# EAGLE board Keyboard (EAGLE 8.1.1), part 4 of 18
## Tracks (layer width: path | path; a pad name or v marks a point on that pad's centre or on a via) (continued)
S$3094 (continued)
  Bottom 0: 16.6,44.39 16.81,44.78
S$3095
  Bottom 0: 16.81,44.78 16.94,45.21
S$3096
  Bottom 0: 16.94,45.21 16.98,45.66
S$3097
  Bottom 0: 16.98,45.66 16.94,46.1
S$3098
  Bottom 0: 16.94,46.1 16.81,46.53
S$3099
  Bottom 0: 16.81,46.53 16.6,46.93
S$3100
  Bottom 0: 16.6,46.93 16.31,47.27
S$3101
  Bottom 0: 16.31,47.27 15.97,47.56
S$3102
  Bottom 0: 15.97,47.56 15.57,47.77
S$3103
  Bottom 0: 15.57,47.77 15.15,47.89
S$3104
  Bottom 0: 15.15,47.89 14.7,47.94
S$3105
  Bottom 0: 14.7,47.94 14.25,47.89
S$3106
  Bottom 0: 14.25,47.89 13.82,47.77
S$3107
  Bottom 0: 13.82,47.77 13.43,47.56
S$3108
  Bottom 0: 13.43,47.56 13.08,47.27
S$3109
  Bottom 0: 13.08,47.27 12.8,46.93
S$3110
  Bottom 0: 12.8,46.93 12.59,46.53
S$3111
  Bottom 0: 12.59,46.53 12.46,46.1
S$3112
  Bottom 0: 12.46,46.1 12.41,45.66
S$3113
  Bottom 0: 12.41,45.66 12.46,45.21
S$3114
  Bottom 0: 12.46,45.21 12.59,44.78
S$3115
  Bottom 0: 12.59,44.78 12.8,44.39
S$3116
  Bottom 0: 12.8,44.39 13.08,44.04
S$3117
  Bottom 0: 13.08,44.04 13.43,43.76
S$3118
  Bottom 0: 13.43,43.76 13.82,43.54
S$3119
  Bottom 0: 13.82,43.54 14.25,43.42
S$3120
  Bottom 0: 14.25,43.42 14.7,43.37
S$3121
  Bottom 0: 9.62,52.8 9.94,52.82
S$3122
  Bottom 0: 9.94,52.82 10.25,52.93
S$3123
  Bottom 0: 10.25,52.93 10.51,53.11
S$3124
  Bottom 0: 10.51,53.11 10.72,53.37
S$3125
  Bottom 0: 10.72,53.37 10.85,53.67
S$3126
  Bottom 0: 10.85,53.67 10.89,53.98
S$3127
  Bottom 0: 10.89,53.98 10.85,54.3
S$3128
  Bottom 0: 10.85,54.3 10.72,54.61
S$3129
  Bottom 0: 10.72,54.61 10.51,54.86
S$3130
  Bottom 0: 10.51,54.86 10.25,55.05
S$3131
  Bottom 0: 10.25,55.05 9.94,55.16
S$3132
  Bottom 0: 9.94,55.16 9.62,55.18
S$3133
  Bottom 0: 9.62,55.18 9.3,55.11
S$3134
  Bottom 0: 9.3,55.11 9.01,54.96
S$3135
  Bottom 0: 9.01,54.96 8.78,54.74
S$3136
  Bottom 0: 8.78,54.74 8.6,54.47
S$3137
  Bottom 0: 8.6,54.47 8.51,54.15
S$3138
  Bottom 0: 8.51,54.15 8.51,53.83
S$3139
  Bottom 0: 8.51,53.83 8.6,53.51
S$3140
  Bottom 0: 8.6,53.51 8.78,53.23
S$3141
  Bottom 0: 8.78,53.23 9.01,53.01
S$3142
  Bottom 0: 9.01,53.01 9.3,52.87
S$3143
  Bottom 0: 9.3,52.87 9.62,52.8
S$3144
  Bottom 0: 9.86,58.23 10.21,58.3
S$3145
  Bottom 0: 10.21,58.3 10.52,58.45
S$3146
  Bottom 0: 10.52,58.45 10.79,58.67
S$3147
  Bottom 0: 10.79,58.67 11,58.96
S$3148
  Bottom 0: 11,58.96 11.13,59.28
S$3149
  Bottom 0: 11.13,59.28 11.17,59.63
S$3150
  Bottom 0: 11.17,59.63 11.13,59.97
S$3151
  Bottom 0: 11.13,59.97 11,60.3
S$3152
  Bottom 0: 11,60.3 10.79,60.58
S$3153
  Bottom 0: 10.79,60.58 10.52,60.8
S$3154
  Bottom 0: 10.52,60.8 10.21,60.96
S$3155
  Bottom 0: 10.21,60.96 9.86,61.02
S$3156
  Bottom 0: 9.86,61.02 9.51,61
S$3157
  Bottom 0: 9.51,61 9.18,60.89
S$3158
  Bottom 0: 9.18,60.89 8.89,60.7
S$3159
  Bottom 0: 8.89,60.7 8.65,60.45
S$3160
  Bottom 0: 8.65,60.45 8.48,60.14
S$3161
  Bottom 0: 8.48,60.14 8.39,59.8
S$3162
  Bottom 0: 8.39,59.8 8.39,59.45
S$3163
  Bottom 0: 8.39,59.45 8.48,59.11
S$3164
  Bottom 0: 8.48,59.11 8.65,58.8
S$3165
  Bottom 0: 8.65,58.8 8.89,58.55
S$3166
  Bottom 0: 8.89,58.55 9.18,58.36
S$3167
  Bottom 0: 9.18,58.36 9.51,58.26
S$3168
  Bottom 0: 9.51,58.26 9.86,58.23
S$3169
  Bottom 0: 10.16,68.64 11.94,68.64
S$3170
  Bottom 0: 11.94,68.64 12.01,68.65
S$3171
  Bottom 0: 12.01,68.65 12.08,68.69
S$3172
  Bottom 0: 12.08,68.69 12.14,68.75
S$3173
  Bottom 0: 12.14,68.75 12.18,68.82
S$3174
  Bottom 0: 12.18,68.82 12.19,68.9
S$3175
  Bottom 0: 12.19,68.9 12.19,70.67
S$3176
  Bottom 0: 12.19,70.67 12.18,70.75
S$3177
  Bottom 0: 12.18,70.75 12.14,70.82
S$3178
  Bottom 0: 12.14,70.82 12.08,70.88
S$3179
  Bottom 0: 12.08,70.88 12.01,70.92
S$3180
  Bottom 0: 12.01,70.92 11.94,70.93
S$3181
  Bottom 0: 11.94,70.93 11.49,70.93
S$3182
  Bottom 0: 11.49,70.93 11.49,71.06
S$3183
  Bottom 0: 11.49,71.06 11.43,71.28
S$3184
  Bottom 0: 11.43,71.28 11.27,71.44
S$3185
  Bottom 0: 11.27,71.44 11.05,71.5
S$3186
  Bottom 0: 11.05,71.5 10.68,71.5
S$3187
  Bottom 0: 10.68,71.5 9.6,72.59
S$3188
  Bottom 0: 9.6,72.59 9.66,72.72
S$3189
  Bottom 0: 9.66,72.72 9.7,73.04
S$3190
  Bottom 0: 9.7,73.04 9.66,73.36
S$3191
  Bottom 0: 9.66,73.36 9.53,73.66
S$3192
  Bottom 0: 9.53,73.66 9.32,73.92
S$3193
  Bottom 0: 9.32,73.92 9.06,74.11
S$3194
  Bottom 0: 9.06,74.11 8.76,74.21
S$3195
  Bottom 0: 8.76,74.21 8.43,74.23
S$3196
  Bottom 0: 8.43,74.23 8.11,74.17
S$3197
  Bottom 0: 8.11,74.17 7.82,74.02
S$3198
  Bottom 0: 7.82,74.02 7.59,73.8
S$3199
  Bottom 0: 7.59,73.8 7.41,73.52
S$3200
  Bottom 0: 7.41,73.52 7.33,73.2
S$3201
  Bottom 0: 7.33,73.2 7.33,72.88
S$3202
  Bottom 0: 7.33,72.88 7.41,72.56
S$3203
  Bottom 0: 7.41,72.56 7.59,72.29
S$3204
  Bottom 0: 7.59,72.29 7.82,72.07
S$3205
  Bottom 0: 7.82,72.07 8.11,71.92
S$3206
  Bottom 0: 8.11,71.92 8.43,71.85
S$3207
  Bottom 0: 8.43,71.85 8.76,71.87
S$3208
  Bottom 0: 8.76,71.87 8.97,71.95
S$3209
  Bottom 0: 8.97,71.95 10.03,70.89
S$3210
  Bottom 0: 10.03,70.89 10.01,70.88
S$3211
  Bottom 0: 10.01,70.88 9.95,70.82
S$3212
  Bottom 0: 9.95,70.82 9.91,70.75
S$3213
  Bottom 0: 9.91,70.75 9.9,70.67
S$3214
  Bottom 0: 9.9,70.67 9.9,68.9
S$3215
  Bottom 0: 9.9,68.9 9.91,68.82
S$3216
  Bottom 0: 9.91,68.82 9.95,68.75
S$3217
  Bottom 0: 9.95,68.75 10.01,68.69
S$3218
  Bottom 0: 10.01,68.69 10.08,68.65
S$3219
  Bottom 0: 10.08,68.65 10.16,68.64
S$3220
  Bottom 0: 39.87,71.85 40.19,71.87
S$3221
  Bottom 0: 40.19,71.87 40.49,71.98
S$3222
  Bottom 0: 40.49,71.98 40.76,72.17
S$3223
  Bottom 0: 40.76,72.17 40.97,72.42
S$3224
  Bottom 0: 40.97,72.42 40.99,72.47
S$3225
  Bottom 0: 40.99,72.47 47.09,72.47
S$3226
  Bottom 0: 47.09,72.47 47.18,72.48
S$3227
  Bottom 0: 47.18,72.48 47.27,72.5
S$3228
  Bottom 0: 47.27,72.5 47.35,72.53
S$3229
  Bottom 0: 47.35,72.53 47.43,72.58
S$3230
  Bottom 0: 47.43,72.58 47.49,72.64
S$3231
  Bottom 0: 47.49,72.64 49.14,74.28
S$3232
  Bottom 0: 49.14,74.28 49.39,74.23
S$3233
  Bottom 0: 49.39,74.23 49.72,74.24
S$3234
  Bottom 0: 49.72,74.24 50.02,74.35
S$3235
  Bottom 0: 50.02,74.35 50.28,74.54
S$3236
  Bottom 0: 50.28,74.54 50.49,74.8
S$3237
  Bottom 0: 50.49,74.8 50.51,74.84
S$3238
  Bottom 0: 50.51,74.84 56.39,74.84
S$3239
  Bottom 0: 56.39,74.84 57.86,73.38
S$3240
  Bottom 0: 57.86,73.38 57.81,73.21
S$3241
  Bottom 0: 57.81,73.21 57.81,72.89
S$3242
  Bottom 0: 57.81,72.89 57.9,72.57
S$3243
  Bottom 0: 57.9,72.57 58.07,72.3
S$3244
  Bottom 0: 58.07,72.3 58.3,72.07
S$3245
  Bottom 0: 58.3,72.07 58.59,71.92
S$3246
  Bottom 0: 58.59,71.92 58.91,71.86
S$3247
  Bottom 0: 58.91,71.86 59.24,71.88
S$3248
  Bottom 0: 59.24,71.88 59.54,71.99
S$3249
  Bottom 0: 59.54,71.99 59.81,72.17
S$3250
  Bottom 0: 59.81,72.17 60.02,72.43
S$3251
  Bottom 0: 60.02,72.43 60.14,72.73
S$3252
  Bottom 0: 60.14,72.73 60.19,73.05
S$3253
  Bottom 0: 60.19,73.05 60.14,73.37
S$3254
  Bottom 0: 60.14,73.37 60.02,73.67
S$3255
  Bottom 0: 60.02,73.67 59.81,73.92
S$3256
  Bottom 0: 59.81,73.92 59.54,74.11
S$3257
  Bottom 0: 59.54,74.11 59.24,74.22
S$3258
  Bottom 0: 59.24,74.22 58.91,74.24
S$3259
  Bottom 0: 58.91,74.24 58.66,74.18
S$3260
  Bottom 0: 58.66,74.18 57.03,75.82
S$3261
  Bottom 0: 57.03,75.82 56.96,75.88
S$3262
  Bottom 0: 56.96,75.88 56.88,75.92
S$3263
  Bottom 0: 56.88,75.92 56.8,75.96
S$3264
  Bottom 0: 56.8,75.96 56.71,75.98
S$3265
  Bottom 0: 56.71,75.98 56.62,75.98
S$3266
  Bottom 0: 56.62,75.98 50.51,75.98
S$3267
  Bottom 0: 50.51,75.98 50.49,76.03
S$3268
  Bottom 0: 50.49,76.03 50.28,76.29
S$3269
  Bottom 0: 50.28,76.29 50.02,76.48
S$3270
  Bottom 0: 50.02,76.48 49.72,76.58
S$3271
  Bottom 0: 49.72,76.58 49.39,76.6
S$3272
  Bottom 0: 49.39,76.6 49.07,76.54
S$3273
  Bottom 0: 49.07,76.54 48.78,76.39
S$3274
  Bottom 0: 48.78,76.39 48.55,76.17
S$3275
  Bottom 0: 48.55,76.17 48.37,75.89
S$3276
  Bottom 0: 48.37,75.89 48.29,75.58
S$3277
  Bottom 0: 48.29,75.58 48.29,75.25
S$3278
  Bottom 0: 48.29,75.25 48.33,75.08
S$3279
  Bottom 0: 48.33,75.08 46.86,73.61
S$3280
  Bottom 0: 46.86,73.61 40.99,73.61
S$3281
  Bottom 0: 40.99,73.61 40.97,73.66
S$3282
  Bottom 0: 40.97,73.66 40.76,73.92
S$3283
  Bottom 0: 40.76,73.92 40.49,74.11
S$3284
  Bottom 0: 40.49,74.11 40.19,74.21
S$3285
  Bottom 0: 40.19,74.21 39.87,74.23
S$3286
  Bottom 0: 39.87,74.23 39.61,74.18
S$3287
  Bottom 0: 39.61,74.18 37.97,75.82
S$3288
  Bottom 0: 37.97,75.82 37.9,75.88
S$3289
  Bottom 0: 37.9,75.88 37.83,75.93
S$3290
  Bottom 0: 37.83,75.93 37.75,75.96
S$3291
  Bottom 0: 37.75,75.96 37.66,75.98
S$3292
  Bottom 0: 37.66,75.98 37.57,75.99
S$3293
  Bottom 0: 37.57,75.99 31.46,75.99
S$3294
  Bottom 0: 31.46,75.99 31.43,76.04
S$3295
  Bottom 0: 31.43,76.04 31.23,76.29
S$3296
  Bottom 0: 31.23,76.29 30.96,76.48
S$3297
  Bottom 0: 30.96,76.48 30.66,76.59
S$3298
  Bottom 0: 30.66,76.59 30.34,76.61
S$3299
  Bottom 0: 30.34,76.61 30.02,76.54
S$3300
  Bottom 0: 30.02,76.54 29.72,76.4
S$3301
  Bottom 0: 29.72,76.4 29.49,76.17
S$3302
  Bottom 0: 29.49,76.17 29.32,75.89
S$3303
  Bottom 0: 29.32,75.89 29.23,75.58
S$3304
  Bottom 0: 29.23,75.58 29.23,75.26
S$3305
  Bottom 0: 29.23,75.26 29.32,74.94
S$3306
  Bottom 0: 29.32,74.94 29.49,74.67
S$3307
  Bottom 0: 29.49,74.67 29.72,74.44
S$3308
  Bottom 0: 29.72,74.44 30.02,74.3
S$3309
  Bottom 0: 30.02,74.3 30.34,74.23
S$3310
  Bottom 0: 30.34,74.23 30.66,74.25
S$3311
  Bottom 0: 30.66,74.25 30.96,74.36
S$3312
  Bottom 0: 30.96,74.36 31.23,74.55
S$3313
  Bottom 0: 31.23,74.55 31.43,74.8
S$3314
  Bottom 0: 31.43,74.8 31.46,74.85
S$3315
  Bottom 0: 31.46,74.85 37.34,74.85
S$3316
  Bottom 0: 37.34,74.85 38.81,73.38
S$3317
  Bottom 0: 38.81,73.38 38.76,73.2
S$3318
  Bottom 0: 38.76,73.2 38.76,72.88
S$3319
  Bottom 0: 38.76,72.88 38.85,72.56
S$3320
  Bottom 0: 38.85,72.56 39.02,72.29
S$3321
  Bottom 0: 39.02,72.29 39.25,72.07
S$3322
  Bottom 0: 39.25,72.07 39.55,71.92
S$3323
  Bottom 0: 39.55,71.92 39.87,71.85
S$3324
  Bottom 0: 232.29,74.23 232.61,74.24
S$3325
  Bottom 0: 232.61,74.24 232.91,74.35
S$3326
  Bottom 0: 232.91,74.35 233.18,74.54
S$3327
  Bottom 0: 233.18,74.54 233.38,74.8
S$3328
  Bottom 0: 233.38,74.8 233.51,75.09
S$3329
  Bottom 0: 233.51,75.09 233.56,75.42
S$3330
  Bottom 0: 233.56,75.42 233.51,75.73
S$3331
  Bottom 0: 233.51,75.73 233.38,76.03
S$3332
  Bottom 0: 233.38,76.03 233.18,76.29
S$3333
  Bottom 0: 233.18,76.29 232.91,76.48
S$3334
  Bottom 0: 232.91,76.48 232.61,76.58
S$3335
  Bottom 0: 232.61,76.58 232.49,76.59
S$3336
  Bottom 0: 232.49,76.59 232.49,77.85
S$3337
  Bottom 0: 232.49,77.85 232.73,77.6
S$3338
  Bottom 0: 232.73,77.6 233.02,77.41
S$3339
  Bottom 0: 233.02,77.41 233.35,77.31
S$3340
  Bottom 0: 233.35,77.31 233.7,77.28
S$3341
  Bottom 0: 233.7,77.28 234.05,77.35
S$3342
  Bottom 0: 234.05,77.35 234.36,77.5
S$3343
  Bottom 0: 234.36,77.5 234.63,77.72
S$3344
  Bottom 0: 234.63,77.72 234.84,78.01
S$3345
  Bottom 0: 234.84,78.01 234.97,78.33
S$3346
  Bottom 0: 234.97,78.33 235.01,78.68
S$3347
  Bottom 0: 235.01,78.68 234.97,79.02
S$3348
  Bottom 0: 234.97,79.02 234.84,79.35
S$3349
  Bottom 0: 234.84,79.35 234.63,79.63
S$3350
  Bottom 0: 234.63,79.63 234.36,79.86
S$3351
  Bottom 0: 234.36,79.86 234.05,80.01
S$3352
  Bottom 0: 234.05,80.01 233.7,80.07
S$3353
  Bottom 0: 233.7,80.07 233.35,80.05
S$3354
  Bottom 0: 233.35,80.05 233.02,79.94
S$3355
  Bottom 0: 233.02,79.94 232.73,79.75
S$3356
  Bottom 0: 232.73,79.75 232.49,79.5
S$3357
  Bottom 0: 232.49,79.5 232.49,84.54
S$3358
  Bottom 0: 232.49,84.54 235.2,87.25
S$3359
  Bottom 0: 235.2,87.25 235.24,87.32
S$3360
  Bottom 0: 235.24,87.32 235.27,87.35
S$3361
  Bottom 0: 235.27,87.35 235.28,87.39
S$3362
  Bottom 0: 235.28,87.39 235.31,87.45
S$3363
  Bottom 0: 235.31,87.45 235.31,87.51
S$3364
  Bottom 0: 235.31,87.51 235.33,87.57
S$3365
  Bottom 0: 235.33,87.57 235.33,87.69
S$3366
  Bottom 0: 235.33,87.69 235.78,87.69
S$3367
  Bottom 0: 235.78,87.69 235.85,87.7
S$3368
  Bottom 0: 235.85,87.7 235.92,87.74
S$3369
  Bottom 0: 235.92,87.74 235.98,87.8
S$3370
  Bottom 0: 235.98,87.8 236.02,87.87
S$3371
  Bottom 0: 236.02,87.87 236.03,87.95
S$3372
  Bottom 0: 236.03,87.95 236.03,89.72
S$3373
  Bottom 0: 236.03,89.72 236.02,89.8
S$3374
  Bottom 0: 236.02,89.8 235.98,89.87
S$3375
  Bottom 0: 235.98,89.87 235.92,89.93
S$3376
  Bottom 0: 235.92,89.93 235.85,89.97
S$3377
  Bottom 0: 235.85,89.97 235.78,89.98
S$3378
  Bottom 0: 235.78,89.98 234,89.98
S$3379
  Bottom 0: 234,89.98 233.92,89.97
S$3380
  Bottom 0: 233.92,89.97 233.85,89.93
S$3381
  Bottom 0: 233.85,89.93 233.79,89.87
S$3382
  Bottom 0: 233.79,89.87 233.75,89.8
S$3383
  Bottom 0: 233.75,89.8 233.74,89.72
S$3384
  Bottom 0: 233.74,89.72 233.74,87.95
S$3385
  Bottom 0: 233.74,87.95 233.75,87.87
S$3386
  Bottom 0: 233.75,87.87 233.79,87.8
S$3387
  Bottom 0: 233.79,87.8 233.85,87.74
S$3388
  Bottom 0: 233.85,87.74 233.92,87.7
S$3389
  Bottom 0: 233.92,87.7 234,87.69
S$3390
  Bottom 0: 234,87.69 234.38,87.69
S$3391
  Bottom 0: 234.38,87.69 231.73,85.05
S$3392
  Bottom 0: 231.73,85.05 231.7,84.99
S$3393
  Bottom 0: 231.7,84.99 231.66,84.93
S$3394
  Bottom 0: 231.66,84.93 231.63,84.87
S$3395
  Bottom 0: 231.63,84.87 231.61,84.8
S$3396
  Bottom 0: 231.61,84.8 231.61,84.73
S$3397
  Bottom 0: 231.61,84.73 231.61,76.33
S$3398
  Bottom 0: 231.61,76.33 231.44,76.17
S$3399
  Bottom 0: 231.44,76.17 231.27,75.89
S$3400
  Bottom 0: 231.27,75.89 231.18,75.58
S$3401
  Bottom 0: 231.18,75.58 231.18,75.25
S$3402
  Bottom 0: 231.18,75.25 231.27,74.94
S$3403
  Bottom 0: 231.27,74.94 231.44,74.66
S$3404
  Bottom 0: 231.44,74.66 231.67,74.44
S$3405
  Bottom 0: 231.67,74.44 231.97,74.29
S$3406
  Bottom 0: 231.97,74.29 232.29,74.23
S$3407
  Bottom 0: 239.91,74.23 240.24,74.24
S$3408
  Bottom 0: 240.24,74.24 240.54,74.35
S$3409
  Bottom 0: 240.54,74.35 240.81,74.54
S$3410
  Bottom 0: 240.81,74.54 241.01,74.8
S$3411
  Bottom 0: 241.01,74.8 241.14,75.09
S$3412
  Bottom 0: 241.14,75.09 241.19,75.42
S$3413
  Bottom 0: 241.19,75.42 241.14,75.73
S$3414
  Bottom 0: 241.14,75.73 241.01,76.03
S$3415
  Bottom 0: 241.01,76.03 240.81,76.29
S$3416
  Bottom 0: 240.81,76.29 240.54,76.48
S$3417
  Bottom 0: 240.54,76.48 240.24,76.58
S$3418
  Bottom 0: 240.24,76.58 239.91,76.6
S$3419
  Bottom 0: 239.91,76.6 239.59,76.54
S$3420
  Bottom 0: 239.59,76.54 239.3,76.39
S$3421
  Bottom 0: 239.3,76.39 239.07,76.17
S$3422
  Bottom 0: 239.07,76.17 238.9,75.89
S$3423
  Bottom 0: 238.9,75.89 238.81,75.58
S$3424
  Bottom 0: 238.81,75.58 238.81,75.25
S$3425
  Bottom 0: 238.81,75.25 238.9,74.94
S$3426
  Bottom 0: 238.9,74.94 239.07,74.66
S$3427
  Bottom 0: 239.07,74.66 239.3,74.44
S$3428
  Bottom 0: 239.3,74.44 239.59,74.29
S$3429
  Bottom 0: 239.59,74.29 239.91,74.23
S$3430
  Bottom 0: 41.77,74.23 42.09,74.24
S$3431
  Bottom 0: 42.09,74.24 42.4,74.35
S$3432
  Bottom 0: 42.4,74.35 42.66,74.54
S$3433
  Bottom 0: 42.66,74.54 42.87,74.8
S$3434
  Bottom 0: 42.87,74.8 43,75.09
S$3435
  Bottom 0: 43,75.09 43.05,75.42
S$3436
  Bottom 0: 43.05,75.42 43,75.73
S$3437
  Bottom 0: 43,75.73 42.87,76.03
S$3438
  Bottom 0: 42.87,76.03 42.66,76.29
S$3439
  Bottom 0: 42.66,76.29 42.4,76.48
S$3440
  Bottom 0: 42.4,76.48 42.09,76.58
S$3441
  Bottom 0: 42.09,76.58 41.98,76.59
S$3442
  Bottom 0: 41.98,76.59 41.98,77.87
S$3443
  Bottom 0: 41.98,77.87 41.99,77.85
S$3444
  Bottom 0: 41.99,77.85 42.23,77.6
S$3445
  Bottom 0: 42.23,77.6 42.52,77.41
S$3446
  Bottom 0: 42.52,77.41 42.85,77.31
S$3447
  Bottom 0: 42.85,77.31 43.2,77.28
S$3448
  Bottom 0: 43.2,77.28 43.55,77.35
S$3449
  Bottom 0: 43.55,77.35 43.86,77.5
S$3450
  Bottom 0: 43.86,77.5 44.13,77.72
S$3451
  Bottom 0: 44.13,77.72 44.34,78.01
S$3452
  Bottom 0: 44.34,78.01 44.47,78.33
S$3453
  Bottom 0: 44.47,78.33 44.51,78.68
S$3454
  Bottom 0: 44.51,78.68 44.47,79.02
S$3455
  Bottom 0: 44.47,79.02 44.34,79.35
S$3456
  Bottom 0: 44.34,79.35 44.13,79.63
S$3457
  Bottom 0: 44.13,79.63 43.86,79.86
S$3458
  Bottom 0: 43.86,79.86 43.55,80.01
S$3459
  Bottom 0: 43.55,80.01 43.2,80.07
S$3460
  Bottom 0: 43.2,80.07 42.85,80.05
S$3461
  Bottom 0: 42.85,80.05 42.52,79.94
S$3462
  Bottom 0: 42.52,79.94 42.23,79.75
S$3463
  Bottom 0: 42.23,79.75 41.99,79.5
S$3464
  Bottom 0: 41.99,79.5 41.98,79.48
S$3465
  Bottom 0: 41.98,79.48 41.98,84.54
S$3466
  Bottom 0: 41.98,84.54 44.7,87.25
S$3467
  Bottom 0: 44.7,87.25 44.73,87.31
S$3468
  Bottom 0: 44.73,87.31 44.77,87.35
S$3469
  Bottom 0: 44.77,87.35 44.78,87.39
S$3470
  Bottom 0: 44.78,87.39 44.81,87.45
S$3471
  Bottom 0: 44.81,87.45 44.81,87.51
S$3472
  Bottom 0: 44.81,87.51 44.83,87.57
S$3473
  Bottom 0: 44.83,87.57 44.83,87.69
S$3474
  Bottom 0: 44.83,87.69 45.28,87.69
S$3475
  Bottom 0: 45.28,87.69 45.35,87.7
S$3476
  Bottom 0: 45.35,87.7 45.42,87.74
S$3477
  Bottom 0: 45.42,87.74 45.48,87.8
S$3478
  Bottom 0: 45.48,87.8 45.52,87.87
S$3479
  Bottom 0: 45.52,87.87 45.53,87.95
S$3480
  Bottom 0: 45.53,87.95 45.53,89.72
S$3481
  Bottom 0: 45.53,89.72 45.52,89.8
S$3482
  Bottom 0: 45.52,89.8 45.48,89.87
S$3483
  Bottom 0: 45.48,89.87 45.42,89.93
S$3484
  Bottom 0: 45.42,89.93 45.35,89.97
S$3485
  Bottom 0: 45.35,89.97 45.28,89.98
S$3486
  Bottom 0: 45.28,89.98 43.5,89.98
S$3487
  Bottom 0: 43.5,89.98 43.42,89.97
S$3488
  Bottom 0: 43.42,89.97 43.35,89.93
S$3489
  Bottom 0: 43.35,89.93 43.29,89.87
S$3490
  Bottom 0: 43.29,89.87 43.25,89.8
S$3491
  Bottom 0: 43.25,89.8 43.24,89.72
S$3492
  Bottom 0: 43.24,89.72 43.24,87.95
S$3493
  Bottom 0: 43.24,87.95 43.25,87.87
S$3494
  Bottom 0: 43.25,87.87 43.29,87.8
S$3495
  Bottom 0: 43.29,87.8 43.35,87.74
S$3496
  Bottom 0: 43.35,87.74 43.42,87.7
S$3497
  Bottom 0: 43.42,87.7 43.5,87.69
S$3498
  Bottom 0: 43.5,87.69 43.89,87.69
S$3499
  Bottom 0: 43.89,87.69 41.22,85.04
S$3500
  Bottom 0: 41.22,85.04 41.18,84.98
S$3501
  Bottom 0: 41.18,84.98 41.15,84.92
S$3502
  Bottom 0: 41.15,84.92 41.12,84.86
S$3503
  Bottom 0: 41.12,84.86 41.1,84.79
S$3504
  Bottom 0: 41.1,84.79 41.09,84.72
S$3505
  Bottom 0: 41.09,84.72 41.09,76.33
S$3506
  Bottom 0: 41.09,76.33 40.93,76.17
S$3507
  Bottom 0: 40.93,76.17 40.75,75.89
S$3508
  Bottom 0: 40.75,75.89 40.67,75.58
S$3509
  Bottom 0: 40.67,75.58 40.67,75.25
S$3510
  Bottom 0: 40.67,75.25 40.75,74.94
S$3511
  Bottom 0: 40.75,74.94 40.93,74.66
S$3512
  Bottom 0: 40.93,74.66 41.16,74.44
S$3513
  Bottom 0: 41.16,74.44 41.45,74.29
S$3514
  Bottom 0: 41.45,74.29 41.77,74.23
S$3515
  Bottom 0: 3.67,74.23 3.99,74.24
S$3516
  Bottom 0: 3.99,74.24 4.29,74.35
S$3517
  Bottom 0: 4.29,74.35 4.56,74.54
S$3518
  Bottom 0: 4.56,74.54 4.76,74.8
S$3519
  Bottom 0: 4.76,74.8 4.89,75.09
S$3520
  Bottom 0: 4.89,75.09 4.94,75.42
S$3521
  Bottom 0: 4.94,75.42 4.89,75.73
S$3522
  Bottom 0: 4.89,75.73 4.76,76.03
S$3523
  Bottom 0: 4.76,76.03 4.56,76.29
S$3524
  Bottom 0: 4.56,76.29 4.29,76.48
S$3525
  Bottom 0: 4.29,76.48 3.99,76.58
S$3526
  Bottom 0: 3.99,76.58 3.88,76.59
S$3527
  Bottom 0: 3.88,76.59 3.88,77.87
S$3528
  Bottom 0: 3.88,77.87 3.89,77.85
S$3529
  Bottom 0: 3.89,77.85 4.13,77.6
S$3530
  Bottom 0: 4.13,77.6 4.42,77.41
S$3531
  Bottom 0: 4.42,77.41 4.75,77.31
S$3532
  Bottom 0: 4.75,77.31 5.1,77.28
S$3533
  Bottom 0: 5.1,77.28 5.45,77.35
S$3534
  Bottom 0: 5.45,77.35 5.76,77.5
S$3535
  Bottom 0: 5.76,77.5 6.03,77.72
S$3536
  Bottom 0: 6.03,77.72 6.24,78.01
S$3537
  Bottom 0: 6.24,78.01 6.37,78.33
S$3538
  Bottom 0: 6.37,78.33 6.41,78.68
S$3539
  Bottom 0: 6.41,78.68 6.37,79.02
S$3540
  Bottom 0: 6.37,79.02 6.24,79.35
S$3541
  Bottom 0: 6.24,79.35 6.03,79.63
S$3542
  Bottom 0: 6.03,79.63 5.76,79.86
S$3543
  Bottom 0: 5.76,79.86 5.45,80.01
S$3544
  Bottom 0: 5.45,80.01 5.1,80.07
S$3545
  Bottom 0: 5.1,80.07 4.75,80.05
S$3546
  Bottom 0: 4.75,80.05 4.42,79.94
S$3547
  Bottom 0: 4.42,79.94 4.13,79.75
S$3548
  Bottom 0: 4.13,79.75 3.89,79.5
S$3549
  Bottom 0: 3.89,79.5 3.88,79.48
S$3550
  Bottom 0: 3.88,79.48 3.88,84.53
S$3551
  Bottom 0: 3.88,84.53 6.6,87.25
S$3552
  Bottom 0: 6.6,87.25 6.64,87.32
S$3553
  Bottom 0: 6.64,87.32 6.67,87.35
S$3554
  Bottom 0: 6.67,87.35 6.68,87.39
S$3555
  Bottom 0: 6.68,87.39 6.71,87.45
S$3556
  Bottom 0: 6.71,87.45 6.71,87.51
S$3557
  Bottom 0: 6.71,87.51 6.73,87.57
S$3558
  Bottom 0: 6.73,87.57 6.73,87.69
S$3559
  Bottom 0: 6.73,87.69 7.18,87.69
S$3560
  Bottom 0: 7.18,87.69 7.25,87.7
S$3561
  Bottom 0: 7.25,87.7 7.32,87.74
S$3562
  Bottom 0: 7.32,87.74 7.38,87.8
S$3563
  Bottom 0: 7.38,87.8 7.42,87.87
S$3564
  Bottom 0: 7.42,87.87 7.43,87.95
S$3565
  Bottom 0: 7.43,87.95 7.43,89.72
S$3566
  Bottom 0: 7.43,89.72 7.42,89.8
S$3567
  Bottom 0: 7.42,89.8 7.38,89.87
S$3568
  Bottom 0: 7.38,89.87 7.32,89.93
S$3569
  Bottom 0: 7.32,89.93 7.25,89.97
S$3570
  Bottom 0: 7.25,89.97 7.18,89.98
S$3571
  Bottom 0: 7.18,89.98 5.4,89.98
S$3572
  Bottom 0: 5.4,89.98 5.32,89.97
S$3573
  Bottom 0: 5.32,89.97 5.25,89.93
S$3574
  Bottom 0: 5.25,89.93 5.19,89.87
S$3575
  Bottom 0: 5.19,89.87 5.15,89.8
S$3576
  Bottom 0: 5.15,89.8 5.14,89.72
S$3577
  Bottom 0: 5.14,89.72 5.14,87.95
S$3578
  Bottom 0: 5.14,87.95 5.15,87.87
S$3579
  Bottom 0: 5.15,87.87 5.19,87.8
S$3580
  Bottom 0: 5.19,87.8 5.25,87.74
S$3581
  Bottom 0: 5.25,87.74 5.32,87.7
S$3582
  Bottom 0: 5.32,87.7 5.4,87.69
S$3583
  Bottom 0: 5.4,87.69 5.78,87.69
S$3584
  Bottom 0: 5.78,87.69 3.12,85.03
S$3585
  Bottom 0: 3.12,85.03 3.08,84.98
S$3586
  Bottom 0: 3.08,84.98 3.04,84.92
S$3587
  Bottom 0: 3.04,84.92 3.02,84.85
S$3588
  Bottom 0: 3.02,84.85 3,84.79
S$3589
  Bottom 0: 3,84.79 3,84.72
S$3590
  Bottom 0: 3,84.72 3,76.33
S$3591
  Bottom 0: 3,76.33 2.82,76.17
S$3592
  Bottom 0: 2.82,76.17 2.65,75.89
S$3593
  Bottom 0: 2.65,75.89 2.56,75.58
S$3594
  Bottom 0: 2.56,75.58 2.56,75.25
S$3595
  Bottom 0: 2.56,75.25 2.65,74.94
S$3596
  Bottom 0: 2.65,74.94 2.82,74.66
S$3597
  Bottom 0: 2.82,74.66 3.05,74.44
S$3598
  Bottom 0: 3.05,74.44 3.35,74.29
S$3599
  Bottom 0: 3.35,74.29 3.67,74.23
S$3600
  Bottom 0: 60.82,74.23 61.15,74.25
S$3601
  Bottom 0: 61.15,74.25 61.45,74.36
S$3602
  Bottom 0: 61.45,74.36 61.71,74.55
S$3603
  Bottom 0: 61.71,74.55 61.92,74.8
S$3604
  Bottom 0: 61.92,74.8 62.05,75.1
S$3605
  Bottom 0: 62.05,75.1 62.09,75.42
S$3606
  Bottom 0: 62.09,75.42 62.05,75.74
S$3607
  Bottom 0: 62.05,75.74 61.92,76.04
S$3608
  Bottom 0: 61.92,76.04 61.71,76.29
S$3609
  Bottom 0: 61.71,76.29 61.45,76.48
S$3610
  Bottom 0: 61.45,76.48 61.15,76.59
S$3611
  Bottom 0: 61.15,76.59 61.03,76.59
S$3612
  Bottom 0: 61.03,76.59 61.03,77.86
S$3613
  Bottom 0: 61.03,77.86 61.04,77.85
S$3614
  Bottom 0: 61.04,77.85 61.28,77.6
S$3615
  Bottom 0: 61.28,77.6 61.57,77.41
S$3616
  Bottom 0: 61.57,77.41 61.9,77.31
S$3617
  Bottom 0: 61.9,77.31 62.25,77.28
S$3618
  Bottom 0: 62.25,77.28 62.6,77.35
S$3619
  Bottom 0: 62.6,77.35 62.91,77.5
S$3620
  Bottom 0: 62.91,77.5 63.18,77.72
S$3621
  Bottom 0: 63.18,77.72 63.39,78.01
S$3622
  Bottom 0: 63.39,78.01 63.52,78.33
S$3623
  Bottom 0: 63.52,78.33 63.56,78.68
S$3624
  Bottom 0: 63.56,78.68 63.52,79.02
S$3625
  Bottom 0: 63.52,79.02 63.39,79.35
S$3626
  Bottom 0: 63.39,79.35 63.18,79.63
S$3627
  Bottom 0: 63.18,79.63 62.91,79.86
S$3628
  Bottom 0: 62.91,79.86 62.6,80.01
S$3629
  Bottom 0: 62.6,80.01 62.25,80.07
S$3630
  Bottom 0: 62.25,80.07 61.9,80.05
S$3631
  Bottom 0: 61.9,80.05 61.57,79.94
S$3632
  Bottom 0: 61.57,79.94 61.28,79.75
S$3633
  Bottom 0: 61.28,79.75 61.04,79.5
S$3634
  Bottom 0: 61.04,79.5 61.03,79.49
S$3635
  Bottom 0: 61.03,79.49 61.03,84.54
S$3636
  Bottom 0: 61.03,84.54 63.75,87.25
S$3637
  Bottom 0: 63.75,87.25 63.78,87.31
S$3638
  Bottom 0: 63.78,87.31 63.82,87.35
S$3639
  Bottom 0: 63.82,87.35 63.83,87.39
S$3640
  Bottom 0: 63.83,87.39 63.86,87.45
S$3641
  Bottom 0: 63.86,87.45 63.86,87.51
S$3642
  Bottom 0: 63.86,87.51 63.88,87.57
S$3643
  Bottom 0: 63.88,87.57 63.88,87.69
S$3644
  Bottom 0: 63.88,87.69 64.33,87.69
S$3645
  Bottom 0: 64.33,87.69 64.4,87.7
S$3646
  Bottom 0: 64.4,87.7 64.47,87.74
S$3647
  Bottom 0: 64.47,87.74 64.53,87.8
S$3648
  Bottom 0: 64.53,87.8 64.57,87.87
S$3649
  Bottom 0: 64.57,87.87 64.58,87.95
S$3650
  Bottom 0: 64.58,87.95 64.58,89.72
S$3651
  Bottom 0: 64.58,89.72 64.57,89.8
S$3652
  Bottom 0: 64.57,89.8 64.53,89.87
S$3653
  Bottom 0: 64.53,89.87 64.47,89.93
S$3654
  Bottom 0: 64.47,89.93 64.4,89.97
S$3655
  Bottom 0: 64.4,89.97 64.33,89.98
S$3656
  Bottom 0: 64.33,89.98 62.55,89.98
S$3657
  Bottom 0: 62.55,89.98 62.47,89.97
S$3658
  Bottom 0: 62.47,89.97 62.4,89.93
S$3659
  Bottom 0: 62.4,89.93 62.34,89.87
S$3660
  Bottom 0: 62.34,89.87 62.3,89.8
S$3661
  Bottom 0: 62.3,89.8 62.29,89.72
S$3662
  Bottom 0: 62.29,89.72 62.29,87.95
S$3663
  Bottom 0: 62.29,87.95 62.3,87.87
S$3664
  Bottom 0: 62.3,87.87 62.34,87.8
S$3665
  Bottom 0: 62.34,87.8 62.4,87.74
S$3666
  Bottom 0: 62.4,87.74 62.47,87.7
S$3667
  Bottom 0: 62.47,87.7 62.55,87.69
S$3668
  Bottom 0: 62.55,87.69 62.94,87.69
S$3669
  Bottom 0: 62.94,87.69 60.28,85.04
S$3670
  Bottom 0: 60.28,85.04 60.23,84.99
S$3671
  Bottom 0: 60.23,84.99 60.2,84.93
S$3672
  Bottom 0: 60.2,84.93 60.17,84.86
S$3673
  Bottom 0: 60.17,84.86 60.16,84.8
S$3674
  Bottom 0: 60.16,84.8 60.15,84.73
S$3675
  Bottom 0: 60.15,84.73 60.15,76.34
S$3676
  Bottom 0: 60.15,76.34 59.98,76.17
S$3677
  Bottom 0: 59.98,76.17 59.8,75.89
S$3678
  Bottom 0: 59.8,75.89 59.72,75.58
S$3679
  Bottom 0: 59.72,75.58 59.72,75.26
S$3680
  Bottom 0: 59.72,75.26 59.8,74.94
S$3681
  Bottom 0: 59.8,74.94 59.98,74.67
S$3682
  Bottom 0: 59.98,74.67 60.21,74.44
S$3683
  Bottom 0: 60.21,74.44 60.5,74.3
S$3684
  Bottom 0: 60.5,74.3 60.82,74.23
S$3685
  Bottom 0: 16.82,78.25 17.34,78.25
S$3686
  Bottom 0: 17.34,78.25 17.85,78.34
S$3687
  Bottom 0: 17.85,78.34 18.34,78.5
S$3688
  Bottom 0: 18.34,78.5 18.79,78.75
S$3689
  Bottom 0: 18.79,78.75 19.2,79.07
S$3690
  Bottom 0: 19.2,79.07 19.55,79.45
S$3691
  Bottom 0: 19.55,79.45 19.84,79.88
S$3692
  Bottom 0: 19.84,79.88 20.05,80.36
S$3693
  Bottom 0: 20.05,80.36 20.18,80.86
S$3694
  Bottom 0: 20.18,80.86 20.21,81.37
S$3695
  Bottom 0: 20.21,81.37 20.18,81.89
S$3696
  Bottom 0: 20.18,81.89 20.05,82.39
S$3697
  Bottom 0: 20.05,82.39 19.84,82.87
S$3698
  Bottom 0: 19.84,82.87 19.55,83.3
S$3699
  Bottom 0: 19.55,83.3 19.2,83.68
S$3700
  Bottom 0: 19.2,83.68 18.79,84
S$3701
  Bottom 0: 18.79,84 18.34,84.24
S$3702
  Bottom 0: 18.34,84.24 17.85,84.41
S$3703
  Bottom 0: 17.85,84.41 17.34,84.5
S$3704
  Bottom 0: 17.34,84.5 16.82,84.5
S$3705
  Bottom 0: 16.82,84.5 16.31,84.41
S$3706
  Bottom 0: 16.31,84.41 15.82,84.24
S$3707
  Bottom 0: 15.82,84.24 15.37,84
S$3708
  Bottom 0: 15.37,84 14.96,83.68
S$3709
  Bottom 0: 14.96,83.68 14.61,83.3
S$3710
  Bottom 0: 14.61,83.3 14.32,82.87
S$3711
  Bottom 0: 14.32,82.87 14.11,82.39
S$3712
  Bottom 0: 14.11,82.39 13.98,81.89
S$3713
  Bottom 0: 13.98,81.89 13.95,81.37
S$3714
  Bottom 0: 13.95,81.37 13.98,80.86
S$3715
  Bottom 0: 13.98,80.86 14.11,80.36
S$3716
  Bottom 0: 14.11,80.36 14.32,79.88
S$3717
  Bottom 0: 14.32,79.88 14.61,79.45
S$3718
  Bottom 0: 14.61,79.45 14.96,79.07
S$3719
  Bottom 0: 14.96,79.07 15.37,78.75
S$3720
  Bottom 0: 15.37,78.75 15.82,78.5
S$3721
  Bottom 0: 15.82,78.5 16.31,78.34
S$3722
  Bottom 0: 16.31,78.34 16.82,78.25
S$3723
  Bottom 0: 55.26,79.17 55.56,79.23
S$3724
  Bottom 0: 55.56,79.23 55.82,79.39
S$3725
  Bottom 0: 55.82,79.39 56.02,79.61
S$3726
  Bottom 0: 56.02,79.61 56.16,79.88
S$3727
  Bottom 0: 56.16,79.88 56.2,80.18
S$3728
  Bottom 0: 56.2,80.18 56.16,80.48
S$3729
  Bottom 0: 56.16,80.48 56.02,80.75
S$3730
  Bottom 0: 56.02,80.75 55.82,80.97
S$3731
  Bottom 0: 55.82,80.97 55.56,81.12
S$3732
  Bottom 0: 55.56,81.12 55.26,81.19
S$3733
  Bottom 0: 55.26,81.19 54.96,81.17
S$3734
  Bottom 0: 54.96,81.17 54.68,81.06
S$3735
  Bottom 0: 54.68,81.06 54.44,80.87
S$3736
  Bottom 0: 54.44,80.87 54.27,80.62
S$3737
  Bottom 0: 54.27,80.62 54.18,80.33
S$3738
  Bottom 0: 54.18,80.33 54.18,80.03
S$3739
  Bottom 0: 54.18,80.03 54.27,79.74
S$3740
  Bottom 0: 54.27,79.74 54.44,79.49
S$3741
  Bottom 0: 54.44,79.49 54.68,79.3
S$3742
  Bottom 0: 54.68,79.3 54.96,79.19
S$3743
  Bottom 0: 54.96,79.19 55.26,79.17
S$3744
  Bottom 0: 207.68,79.17 207.97,79.24
S$3745
  Bottom 0: 207.97,79.24 208.24,79.39
S$3746
  Bottom 0: 208.24,79.39 208.44,79.61
S$3747
  Bottom 0: 208.44,79.61 208.57,79.89
S$3748
  Bottom 0: 208.57,79.89 208.62,80.19
S$3749
  Bottom 0: 208.62,80.19 208.57,80.48
S$3750
  Bottom 0: 208.57,80.48 208.44,80.76
S$3751
  Bottom 0: 208.44,80.76 208.24,80.98
S$3752
  Bottom 0: 208.24,80.98 207.97,81.13
S$3753
  Bottom 0: 207.97,81.13 207.68,81.2
S$3754
  Bottom 0: 207.68,81.2 207.37,81.18
S$3755
  Bottom 0: 207.37,81.18 207.09,81.06
S$3756
  Bottom 0: 207.09,81.06 206.85,80.88
S$3757
  Bottom 0: 206.85,80.88 206.69,80.63
S$3758
  Bottom 0: 206.69,80.63 206.59,80.34
S$3759
  Bottom 0: 206.59,80.34 206.59,80.03
S$3760
  Bottom 0: 206.59,80.03 206.69,79.74
S$3761
  Bottom 0: 206.69,79.74 206.85,79.49
S$3762
  Bottom 0: 206.85,79.49 207.09,79.31
S$3763
  Bottom 0: 207.09,79.31 207.37,79.19
S$3764
  Bottom 0: 207.37,79.19 207.68,79.17
S$3765
  Bottom 0: 68.6,79.83 68.95,79.89
S$3766
  Bottom 0: 68.95,79.89 69.26,80.04
S$3767
  Bottom 0: 69.26,80.04 69.53,80.26
S$3768
  Bottom 0: 69.53,80.26 69.74,80.55
S$3769
  Bottom 0: 69.74,80.55 69.87,80.87
S$3770
  Bottom 0: 69.87,80.87 69.91,81.22
S$3771
  Bottom 0: 69.91,81.22 69.87,81.56
S$3772
  Bottom 0: 69.87,81.56 69.74,81.89
S$3773
  Bottom 0: 69.74,81.89 69.53,82.17
S$3774
  Bottom 0: 69.53,82.17 69.26,82.39
S$3775
  Bottom 0: 69.26,82.39 68.95,82.55
S$3776
  Bottom 0: 68.95,82.55 68.6,82.61
S$3777
  Bottom 0: 68.6,82.61 68.25,82.59
S$3778
  Bottom 0: 68.25,82.59 67.92,82.48
S$3779
  Bottom 0: 67.92,82.48 67.63,82.29
S$3780
  Bottom 0: 67.63,82.29 67.39,82.04
S$3781
  Bottom 0: 67.39,82.04 67.22,81.73
S$3782
  Bottom 0: 67.22,81.73 67.13,81.39
S$3783
  Bottom 0: 67.13,81.39 67.13,81.04
S$3784
  Bottom 0: 67.13,81.04 67.22,80.7
S$3785
  Bottom 0: 67.22,80.7 67.39,80.39
S$3786
  Bottom 0: 67.39,80.39 67.63,80.14
S$3787
  Bottom 0: 67.63,80.14 67.92,79.95
S$3788
  Bottom 0: 67.92,79.95 68.25,79.84
S$3789
  Bottom 0: 68.25,79.84 68.6,79.83
S$3790
  Bottom 0: 49.55,79.83 49.9,79.89
S$3791
  Bottom 0: 49.9,79.89 50.21,80.04
S$3792
  Bottom 0: 50.21,80.04 50.48,80.26
S$3793
  Bottom 0: 50.48,80.26 50.69,80.55
S$3794
  Bottom 0: 50.69,80.55 50.82,80.87
S$3795
  Bottom 0: 50.82,80.87 50.86,81.22
S$3796
  Bottom 0: 50.86,81.22 50.82,81.56
S$3797
  Bottom 0: 50.82,81.56 50.69,81.89
S$3798
  Bottom 0: 50.69,81.89 50.48,82.17
S$3799
  Bottom 0: 50.48,82.17 50.21,82.39
S$3800
  Bottom 0: 50.21,82.39 49.9,82.55
S$3801
  Bottom 0: 49.9,82.55 49.55,82.61
S$3802
  Bottom 0: 49.55,82.61 49.2,82.59
S$3803
  Bottom 0: 49.2,82.59 48.87,82.48
S$3804
  Bottom 0: 48.87,82.48 48.58,82.29
S$3805
  Bottom 0: 48.58,82.29 48.34,82.04
S$3806
  Bottom 0: 48.34,82.04 48.17,81.73
S$3807
  Bottom 0: 48.17,81.73 48.08,81.39
S$3808
  Bottom 0: 48.08,81.39 48.08,81.04
S$3809
  Bottom 0: 48.08,81.04 48.17,80.7
S$3810
  Bottom 0: 48.17,80.7 48.34,80.39
S$3811
  Bottom 0: 48.34,80.39 48.58,80.14
S$3812
  Bottom 0: 48.58,80.14 48.87,79.95
S$3813
  Bottom 0: 48.87,79.95 49.2,79.84
S$3814
  Bottom 0: 49.2,79.84 49.55,79.83
S$3815
  Bottom 0: 236.16,81.47 236.6,81.52
S$3816
  Bottom 0: 236.6,81.52 237.03,81.64
S$3817
  Bottom 0: 237.03,81.64 237.43,81.86
S$3818
  Bottom 0: 237.43,81.86 237.77,82.14
S$3819
  Bottom 0: 237.77,82.14 238.06,82.49
S$3820
  Bottom 0: 238.06,82.49 238.27,82.88
S$3821
  Bottom 0: 238.27,82.88 238.4,83.31
S$3822
  Bottom 0: 238.4,83.31 238.44,83.76
S$3823
  Bottom 0: 238.44,83.76 238.4,84.2
S$3824
  Bottom 0: 238.4,84.2 238.27,84.63
S$3825
  Bottom 0: 238.27,84.63 238.06,85.03
S$3826
  Bottom 0: 238.06,85.03 237.77,85.37
S$3827
  Bottom 0: 237.77,85.37 237.43,85.66
S$3828
  Bottom 0: 237.43,85.66 237.03,85.87
S$3829
  Bottom 0: 237.03,85.87 236.6,86
S$3830
  Bottom 0: 236.6,86 236.16,86.04
S$3831
  Bottom 0: 236.16,86.04 235.71,86
S$3832
  Bottom 0: 235.71,86 235.28,85.87
S$3833
  Bottom 0: 235.28,85.87 234.89,85.66
S$3834
  Bottom 0: 234.89,85.66 234.54,85.37
S$3835
  Bottom 0: 234.54,85.37 234.26,85.03
S$3836
  Bottom 0: 234.26,85.03 234.04,84.63
S$3837
  Bottom 0: 234.04,84.63 233.92,84.2
S$3838
  Bottom 0: 233.92,84.2 233.87,83.76
S$3839
  Bottom 0: 233.87,83.76 233.92,83.31
S$3840
  Bottom 0: 233.92,83.31 234.04,82.88
S$3841
  Bottom 0: 234.04,82.88 234.26,82.49
S$3842
  Bottom 0: 234.26,82.49 234.54,82.14
S$3843
  Bottom 0: 234.54,82.14 234.89,81.86
S$3844
  Bottom 0: 234.89,81.86 235.28,81.64
S$3845
  Bottom 0: 235.28,81.64 235.71,81.52
S$3846
  Bottom 0: 235.71,81.52 236.16,81.47
S$3847
  Bottom 0: 179.01,81.47 179.45,81.52
S$3848
  Bottom 0: 179.45,81.52 179.88,81.64
S$3849
  Bottom 0: 179.88,81.64 180.28,81.86
S$3850
  Bottom 0: 180.28,81.86 180.62,82.14
S$3851
  Bottom 0: 180.62,82.14 180.91,82.49
S$3852
  Bottom 0: 180.91,82.49 181.12,82.88
S$3853
  Bottom 0: 181.12,82.88 181.25,83.31
S$3854
  Bottom 0: 181.25,83.31 181.29,83.76
S$3855
  Bottom 0: 181.29,83.76 181.25,84.2
S$3856
  Bottom 0: 181.25,84.2 181.12,84.63
S$3857
  Bottom 0: 181.12,84.63 180.91,85.03
S$3858
  Bottom 0: 180.91,85.03 180.62,85.37
S$3859
  Bottom 0: 180.62,85.37 180.28,85.66
S$3860
  Bottom 0: 180.28,85.66 179.88,85.87
S$3861
  Bottom 0: 179.88,85.87 179.45,86
S$3862
  Bottom 0: 179.45,86 179.01,86.04
S$3863
  Bottom 0: 179.01,86.04 178.56,86
S$3864
  Bottom 0: 178.56,86 178.13,85.87
S$3865
  Bottom 0: 178.13,85.87 177.74,85.66
S$3866
  Bottom 0: 177.74,85.66 177.39,85.37
S$3867
  Bottom 0: 177.39,85.37 177.11,85.03
S$3868
  Bottom 0: 177.11,85.03 176.89,84.63
S$3869
  Bottom 0: 176.89,84.63 176.77,84.2
S$3870
  Bottom 0: 176.77,84.2 176.72,83.76
S$3871
  Bottom 0: 176.72,83.76 176.77,83.31
S$3872
  Bottom 0: 176.77,83.31 176.89,82.88
S$3873
  Bottom 0: 176.89,82.88 177.11,82.49
S$3874
  Bottom 0: 177.11,82.49 177.39,82.14
S$3875
  Bottom 0: 177.39,82.14 177.74,81.86
S$3876
  Bottom 0: 177.74,81.86 178.13,81.64
S$3877
  Bottom 0: 178.13,81.64 178.56,81.52
S$3878
  Bottom 0: 178.56,81.52 179.01,81.47
S$3879
  Bottom 0: 64.71,81.47 65.15,81.52
S$3880
  Bottom 0: 65.15,81.52 65.58,81.64
S$3881
  Bottom 0: 65.58,81.64 65.98,81.86
S$3882
  Bottom 0: 65.98,81.86 66.32,82.14
S$3883
  Bottom 0: 66.32,82.14 66.61,82.49
S$3884
  Bottom 0: 66.61,82.49 66.82,82.88
S$3885
  Bottom 0: 66.82,82.88 66.95,83.31
S$3886
  Bottom 0: 66.95,83.31 66.99,83.76
S$3887
  Bottom 0: 66.99,83.76 66.95,84.2
S$3888
  Bottom 0: 66.95,84.2 66.82,84.63
S$3889
  Bottom 0: 66.82,84.63 66.61,85.03
S$3890
  Bottom 0: 66.61,85.03 66.32,85.37
S$3891
  Bottom 0: 66.32,85.37 65.98,85.66
S$3892
  Bottom 0: 65.98,85.66 65.58,85.87
S$3893
  Bottom 0: 65.58,85.87 65.15,86
S$3894
  Bottom 0: 65.15,86 64.71,86.04
S$3895
  Bottom 0: 64.71,86.04 64.26,86
S$3896
  Bottom 0: 64.26,86 63.83,85.87
S$3897
  Bottom 0: 63.83,85.87 63.44,85.66
S$3898
  Bottom 0: 63.44,85.66 63.09,85.37
S$3899
  Bottom 0: 63.09,85.37 62.81,85.03
S$3900
  Bottom 0: 62.81,85.03 62.59,84.63
S$3901
  Bottom 0: 62.59,84.63 62.46,84.2
S$3902
  Bottom 0: 62.46,84.2 62.42,83.76
S$3903
  Bottom 0: 62.42,83.76 62.46,83.31
S$3904
  Bottom 0: 62.46,83.31 62.59,82.88
S$3905
  Bottom 0: 62.59,82.88 62.81,82.49
S$3906
  Bottom 0: 62.81,82.49 63.09,82.14
S$3907
  Bottom 0: 63.09,82.14 63.44,81.86
S$3908
  Bottom 0: 63.44,81.86 63.83,81.64
S$3909
  Bottom 0: 63.83,81.64 64.26,81.52
S$3910
  Bottom 0: 64.26,81.52 64.71,81.47
S$3911
  Bottom 0: 45.66,81.47 46.1,81.52
S$3912
  Bottom 0: 46.1,81.52 46.53,81.64
S$3913
  Bottom 0: 46.53,81.64 46.93,81.86
S$3914
  Bottom 0: 46.93,81.86 47.27,82.14
S$3915
  Bottom 0: 47.27,82.14 47.56,82.49
S$3916
  Bottom 0: 47.56,82.49 47.77,82.88
S$3917
  Bottom 0: 47.77,82.88 47.9,83.31
S$3918
  Bottom 0: 47.9,83.31 47.94,83.76
S$3919
  Bottom 0: 47.94,83.76 47.9,84.2
S$3920
  Bottom 0: 47.9,84.2 47.77,84.63
S$3921
  Bottom 0: 47.77,84.63 47.56,85.03
S$3922
  Bottom 0: 47.56,85.03 47.27,85.37
S$3923
  Bottom 0: 47.27,85.37 46.93,85.66
S$3924
  Bottom 0: 46.93,85.66 46.53,85.87
S$3925
  Bottom 0: 46.53,85.87 46.1,86
S$3926
  Bottom 0: 46.1,86 45.66,86.04
S$3927
  Bottom 0: 45.66,86.04 45.21,86
S$3928
  Bottom 0: 45.21,86 44.78,85.87
S$3929
  Bottom 0: 44.78,85.87 44.39,85.66
S$3930
  Bottom 0: 44.39,85.66 44.04,85.37
S$3931
  Bottom 0: 44.04,85.37 43.76,85.03
S$3932
  Bottom 0: 43.76,85.03 43.54,84.63
S$3933
  Bottom 0: 43.54,84.63 43.41,84.2
S$3934
  Bottom 0: 43.41,84.2 43.37,83.76
S$3935
  Bottom 0: 43.37,83.76 43.41,83.31
S$3936
  Bottom 0: 43.41,83.31 43.54,82.88
S$3937
  Bottom 0: 43.54,82.88 43.76,82.49
S$3938
  Bottom 0: 43.76,82.49 44.04,82.14
S$3939
  Bottom 0: 44.04,82.14 44.39,81.86
S$3940
  Bottom 0: 44.39,81.86 44.78,81.64
S$3941
  Bottom 0: 44.78,81.64 45.21,81.52
S$3942
  Bottom 0: 45.21,81.52 45.66,81.47
S$3943
  Bottom 0: 55.26,86.79 55.56,86.86
S$3944
  Bottom 0: 55.56,86.86 55.82,87.01
S$3945
  Bottom 0: 55.82,87.01 56.02,87.23
S$3946
  Bottom 0: 56.02,87.23 56.16,87.5
S$3947
  Bottom 0: 56.16,87.5 56.2,87.8
S$3948
  Bottom 0: 56.2,87.8 56.16,88.1
S$3949
  Bottom 0: 56.16,88.1 56.02,88.37
S$3950
  Bottom 0: 56.02,88.37 55.82,88.59
S$3951
  Bottom 0: 55.82,88.59 55.56,88.75
S$3952
  Bottom 0: 55.56,88.75 55.26,88.81
S$3953
  Bottom 0: 55.26,88.81 54.96,88.79
S$3954
  Bottom 0: 54.96,88.79 54.68,88.68
S$3955
  Bottom 0: 54.68,88.68 54.44,88.49
S$3956
  Bottom 0: 54.44,88.49 54.27,88.24
S$3957
  Bottom 0: 54.27,88.24 54.18,87.95
S$3958
  Bottom 0: 54.18,87.95 54.18,87.65
S$3959
  Bottom 0: 54.18,87.65 54.27,87.36
S$3960
  Bottom 0: 54.27,87.36 54.44,87.11
S$3961
  Bottom 0: 54.44,87.11 54.68,86.92
S$3962
  Bottom 0: 54.68,86.92 54.96,86.81
S$3963
  Bottom 0: 54.96,86.81 55.26,86.79
S$3964
  Bottom 0: 226.73,86.79 227.02,86.86
S$3965
  Bottom 0: 227.02,86.86 227.29,87.01
S$3966
  Bottom 0: 227.29,87.01 227.49,87.23
S$3967
  Bottom 0: 227.49,87.23 227.62,87.51
S$3968
  Bottom 0: 227.62,87.51 227.67,87.81
S$3969
  Bottom 0: 227.67,87.81 227.62,88.11
S$3970
  Bottom 0: 227.62,88.11 227.49,88.38
S$3971
  Bottom 0: 227.49,88.38 227.29,88.6
S$3972
  Bottom 0: 227.29,88.6 227.02,88.75
S$3973
  Bottom 0: 227.02,88.75 226.73,88.82
S$3974
  Bottom 0: 226.73,88.82 226.42,88.8
S$3975
  Bottom 0: 226.42,88.8 226.14,88.68
S$3976
  Bottom 0: 226.14,88.68 225.91,88.5
S$3977
  Bottom 0: 225.91,88.5 225.74,88.25
S$3978
  Bottom 0: 225.74,88.25 225.64,87.96
S$3979
  Bottom 0: 225.64,87.96 225.64,87.65
S$3980
  Bottom 0: 225.64,87.65 225.74,87.36
S$3981
  Bottom 0: 225.74,87.36 225.91,87.11
S$3982
  Bottom 0: 225.91,87.11 226.14,86.93
S$3983
  Bottom 0: 226.14,86.93 226.42,86.81
S$3984
  Bottom 0: 226.42,86.81 226.73,86.79
S$3985
  Bottom 0: 207.68,86.79 207.97,86.86
S$3986
  Bottom 0: 207.97,86.86 208.24,87.01
S$3987
  Bottom 0: 208.24,87.01 208.44,87.23
S$3988
  Bottom 0: 208.44,87.23 208.57,87.51
S$3989
  Bottom 0: 208.57,87.51 208.62,87.81
S$3990
  Bottom 0: 208.62,87.81 208.57,88.11
S$3991
  Bottom 0: 208.57,88.11 208.44,88.38
S$3992
  Bottom 0: 208.44,88.38 208.24,88.6
S$3993
  Bottom 0: 208.24,88.6 207.97,88.75
S$3994
  Bottom 0: 207.97,88.75 207.68,88.82
S$3995
  Bottom 0: 207.68,88.82 207.37,88.8
S$3996
  Bottom 0: 207.37,88.8 207.09,88.68
S$3997
  Bottom 0: 207.09,88.68 206.85,88.5
S$3998
  Bottom 0: 206.85,88.5 206.69,88.25
S$3999
  Bottom 0: 206.69,88.25 206.59,87.96
S$4000
  Bottom 0: 206.59,87.96 206.59,87.65
S$4001
  Bottom 0: 206.59,87.65 206.69,87.36
S$4002
  Bottom 0: 206.69,87.36 206.85,87.11
S$4003
  Bottom 0: 206.85,87.11 207.09,86.93
S$4004
  Bottom 0: 207.09,86.93 207.37,86.81
S$4005
  Bottom 0: 207.37,86.81 207.68,86.79
S$4006
  Bottom 0: 187.44,86.79 187.73,86.86
S$4007
  Bottom 0: 187.73,86.86 188,87.01
S$4008
  Bottom 0: 188,87.01 188.2,87.23
S$4009
  Bottom 0: 188.2,87.23 188.33,87.51
S$4010
  Bottom 0: 188.33,87.51 188.38,87.81
S$4011
  Bottom 0: 188.38,87.81 188.33,88.11
S$4012
  Bottom 0: 188.33,88.11 188.2,88.38
S$4013
  Bottom 0: 188.2,88.38 188,88.6
S$4014
  Bottom 0: 188,88.6 187.73,88.75
S$4015
  Bottom 0: 187.73,88.75 187.44,88.82
S$4016
  Bottom 0: 187.44,88.82 187.13,88.8
S$4017
  Bottom 0: 187.13,88.8 186.85,88.68
S$4018
  Bottom 0: 186.85,88.68 186.62,88.5
S$4019
  Bottom 0: 186.62,88.5 186.45,88.25
S$4020
  Bottom 0: 186.45,88.25 186.36,87.96
S$4021
  Bottom 0: 186.36,87.96 186.36,87.65
S$4022
  Bottom 0: 186.36,87.65 186.45,87.36
S$4023
  Bottom 0: 186.45,87.36 186.62,87.11
S$4024
  Bottom 0: 186.62,87.11 186.85,86.93
S$4025
  Bottom 0: 186.85,86.93 187.13,86.81
S$4026
  Bottom 0: 187.13,86.81 187.44,86.79
S$4027
  Bottom 0: 75.51,86.79 75.8,86.86
S$4028
  Bottom 0: 75.8,86.86 76.06,87.01
S$4029
  Bottom 0: 76.06,87.01 76.27,87.23
S$4030
  Bottom 0: 76.27,87.23 76.4,87.51
S$4031
  Bottom 0: 76.4,87.51 76.45,87.81
S$4032
  Bottom 0: 76.45,87.81 76.4,88.11
S$4033
  Bottom 0: 76.4,88.11 76.27,88.38
S$4034
  Bottom 0: 76.27,88.38 76.06,88.6
S$4035
  Bottom 0: 76.06,88.6 75.8,88.75
S$4036
  Bottom 0: 75.8,88.75 75.51,88.82
S$4037
  Bottom 0: 75.51,88.82 75.2,88.8
S$4038
  Bottom 0: 75.2,88.8 74.92,88.68
S$4039
  Bottom 0: 74.92,88.68 74.68,88.5
S$4040
  Bottom 0: 74.68,88.5 74.52,88.25
S$4041
  Bottom 0: 74.52,88.25 74.42,87.96
S$4042
  Bottom 0: 74.42,87.96 74.42,87.65
S$4043
  Bottom 0: 74.42,87.65 74.52,87.36
S$4044
  Bottom 0: 74.52,87.36 74.68,87.11
S$4045
  Bottom 0: 74.68,87.11 74.92,86.93
S$4046
  Bottom 0: 74.92,86.93 75.2,86.81
S$4047
  Bottom 0: 75.2,86.81 75.51,86.79
S$4048
  Bottom 0: 37.4,86.79 37.69,86.86
S$4049
  Bottom 0: 37.69,86.86 37.96,87.01
S$4050
  Bottom 0: 37.96,87.01 38.16,87.23
S$4051
  Bottom 0: 38.16,87.23 38.29,87.51
S$4052
  Bottom 0: 38.29,87.51 38.34,87.81
S$4053
  Bottom 0: 38.34,87.81 38.29,88.11
S$4054
  Bottom 0: 38.29,88.11 38.16,88.38
S$4055
  Bottom 0: 38.16,88.38 37.96,88.6
S$4056
  Bottom 0: 37.96,88.6 37.69,88.75
S$4057
  Bottom 0: 37.69,88.75 37.4,88.82
S$4058
  Bottom 0: 37.4,88.82 37.09,88.8
S$4059
  Bottom 0: 37.09,88.8 36.82,88.68
S$4060
  Bottom 0: 36.82,88.68 36.58,88.5
S$4061
  Bottom 0: 36.58,88.5 36.41,88.25
S$4062
  Bottom 0: 36.41,88.25 36.32,87.96
S$4063
  Bottom 0: 36.32,87.96 36.32,87.65
S$4064
  Bottom 0: 36.32,87.65 36.41,87.36
S$4065
  Bottom 0: 36.41,87.36 36.58,87.11
S$4066
  Bottom 0: 36.58,87.11 36.82,86.93
S$4067
  Bottom 0: 36.82,86.93 37.09,86.81
S$4068
  Bottom 0: 37.09,86.81 37.4,86.79
S$4069
  Bottom 0: 35.02,86.79 35.32,86.86
S$4070
  Bottom 0: 35.32,86.86 35.58,87.01
S$4071
  Bottom 0: 35.58,87.01 35.78,87.23
S$4072
  Bottom 0: 35.78,87.23 35.92,87.51
S$4073
  Bottom 0: 35.92,87.51 35.96,87.81
S$4074
  Bottom 0: 35.96,87.81 35.92,88.11
S$4075
  Bottom 0: 35.92,88.11 35.78,88.38
S$4076
  Bottom 0: 35.78,88.38 35.58,88.6
S$4077
  Bottom 0: 35.58,88.6 35.32,88.75
S$4078
  Bottom 0: 35.32,88.75 35.02,88.82
S$4079
  Bottom 0: 35.02,88.82 34.72,88.8
S$4080
  Bottom 0: 34.72,88.8 34.44,88.68
S$4081
  Bottom 0: 34.44,88.68 34.2,88.5
S$4082
  Bottom 0: 34.2,88.5 34.03,88.25
S$4083
  Bottom 0: 34.03,88.25 33.94,87.96
S$4084
  Bottom 0: 33.94,87.96 33.94,87.65
S$4085
  Bottom 0: 33.94,87.65 34.03,87.36
S$4086
  Bottom 0: 34.03,87.36 34.2,87.11
S$4087
  Bottom 0: 34.2,87.11 34.44,86.93
S$4088
  Bottom 0: 34.44,86.93 34.72,86.81
S$4089
  Bottom 0: 34.72,86.81 35.02,86.79
S$4090
  Bottom 0: 281.99,87.25 281.99,87.95
S$4091
  Bottom 0: 281.99,87.95 281.29,87.95
S$4092
  Bottom 0: 281.29,87.95 281.43,87.7
S$4093
  Bottom 0: 281.43,87.7 281.67,87.44
S$4094
  Bottom 0: 281.67,87.44 281.96,87.26
S$4095
  Bottom 0: 281.96,87.26 281.99,87.25
S$4096
  Bottom 0: 283.14,87.26 283.31,87.34
S$4097
  Bottom 0: 283.31,87.34 283.58,87.57
S$4098
  Bottom 0: 283.58,87.57 283.79,87.85
S$4099
  Bottom 0: 283.79,87.85 283.83,87.95
S$4100
  Bottom 0: 283.83,87.95 283.14,87.95
S$4101
  Bottom 0: 283.14,87.95 283.14,87.26
S$4102
  Bottom 0: 65.81,87.7 66.14,87.7
S$4103
  Bottom 0: 66.14,87.7 66.45,87.8
S$4104
  Bottom 0: 66.45,87.8 66.72,87.97
S$4105
  Bottom 0: 66.72,87.97 66.93,88.22
S$4106
  Bottom 0: 66.93,88.22 67.07,88.52
S$4107
  Bottom 0: 67.07,88.52 67.12,88.84
S$4108
  Bottom 0: 67.12,88.84 67.07,89.16
S$4109
  Bottom 0: 67.07,89.16 66.93,89.46
S$4110
  Bottom 0: 66.93,89.46 66.72,89.7
S$4111
  Bottom 0: 66.72,89.7 66.45,89.88
S$4112
  Bottom 0: 66.45,89.88 66.14,89.97
S$4113
  Bottom 0: 66.14,89.97 65.81,89.97
S$4114
  Bottom 0: 65.81,89.97 65.5,89.88
S$4115
  Bottom 0: 65.5,89.88 65.23,89.7
S$4116
  Bottom 0: 65.23,89.7 65.02,89.46
S$4117
  Bottom 0: 65.02,89.46 64.88,89.16
S$4118
  Bottom 0: 64.88,89.16 64.83,88.84
S$4119
  Bottom 0: 64.83,88.84 64.88,88.52
S$4120
  Bottom 0: 64.88,88.52 65.02,88.22
S$4121
  Bottom 0: 65.02,88.22 65.23,87.97
S$4122
  Bottom 0: 65.23,87.97 65.5,87.8
S$4123
  Bottom 0: 65.5,87.8 65.81,87.7
S$4124
  Bottom 0: 46.76,87.7 47.09,87.7
S$4125
  Bottom 0: 47.09,87.7 47.4,87.8
S$4126
  Bottom 0: 47.4,87.8 47.67,87.97
S$4127
  Bottom 0: 47.67,87.97 47.88,88.22
S$4128
  Bottom 0: 47.88,88.22 48.02,88.52
S$4129
  Bottom 0: 48.02,88.52 48.07,88.84
S$4130
  Bottom 0: 48.07,88.84 48.02,89.16
S$4131
  Bottom 0: 48.02,89.16 47.88,89.46
S$4132
  Bottom 0: 47.88,89.46 47.67,89.7
S$4133
  Bottom 0: 47.67,89.7 47.4,89.88
S$4134
  Bottom 0: 47.4,89.88 47.09,89.97
S$4135
  Bottom 0: 47.09,89.97 46.76,89.97
S$4136
  Bottom 0: 46.76,89.97 46.45,89.88
S$4137
  Bottom 0: 46.45,89.88 46.18,89.7
S$4138
  Bottom 0: 46.18,89.7 45.97,89.46
S$4139
  Bottom 0: 45.97,89.46 45.83,89.16
S$4140
  Bottom 0: 45.83,89.16 45.78,88.84
S$4141
  Bottom 0: 45.78,88.84 45.83,88.52
S$4142
  Bottom 0: 45.83,88.52 45.97,88.22
S$4143
  Bottom 0: 45.97,88.22 46.18,87.97
S$4144
  Bottom 0: 46.18,87.97 46.45,87.8
S$4145
  Bottom 0: 46.45,87.8 46.76,87.7
S$4146
  Bottom 0: 27.71,87.7 28.04,87.7
S$4147
  Bottom 0: 28.04,87.7 28.35,87.8
S$4148
  Bottom 0: 28.35,87.8 28.62,87.97
S$4149
  Bottom 0: 28.62,87.97 28.83,88.22
S$4150
  Bottom 0: 28.83,88.22 28.97,88.52
S$4151
  Bottom 0: 28.97,88.52 29.02,88.84
S$4152
  Bottom 0: 29.02,88.84 28.97,89.16
S$4153
  Bottom 0: 28.97,89.16 28.83,89.46
S$4154
  Bottom 0: 28.83,89.46 28.62,89.7
S$4155
  Bottom 0: 28.62,89.7 28.35,89.88
S$4156
  Bottom 0: 28.35,89.88 28.04,89.97
S$4157
  Bottom 0: 28.04,89.97 27.71,89.97
S$4158
  Bottom 0: 27.71,89.97 27.4,89.88
S$4159
  Bottom 0: 27.4,89.88 27.13,89.7
S$4160
  Bottom 0: 27.13,89.7 26.92,89.46
S$4161
  Bottom 0: 26.92,89.46 26.78,89.16
S$4162
  Bottom 0: 26.78,89.16 26.73,88.84
S$4163
  Bottom 0: 26.73,88.84 26.78,88.52
S$4164
  Bottom 0: 26.78,88.52 26.92,88.22
S$4165
  Bottom 0: 26.92,88.22 27.13,87.97
S$4166
  Bottom 0: 27.13,87.97 27.4,87.8
S$4167
  Bottom 0: 27.4,87.8 27.71,87.7
S$4168
  Bottom 0: 283.14,89.1 283.83,89.1
S$4169
  Bottom 0: 283.83,89.1 283.79,89.2
S$4170
  Bottom 0: 283.79,89.2 283.58,89.49
S$4171
  Bottom 0: 283.58,89.49 283.31,89.71
S$4172
  Bottom 0: 283.31,89.71 283.14,89.79
S$4173
  Bottom 0: 283.14,89.79 283.14,89.1
S$4174
  Bottom 0: 281.29,89.1 281.99,89.1
S$4175
  Bottom 0: 281.99,89.1 281.99,89.81
S$4176
  Bottom 0: 281.99,89.81 281.96,89.8
S$4177
  Bottom 0: 281.96,89.8 281.67,89.61
S$4178
  Bottom 0: 281.67,89.61 281.43,89.35
S$4179
  Bottom 0: 281.43,89.35 281.29,89.1
S$4180
  Bottom 0: 18.42,1.99 18.43,1.99
S$4181
  Bottom 0: 18.43,1.99 18.64,2.21
S$4182
  Bottom 0: 18.64,2.21 18.7,2.34
S$4183
  Bottom 0: 18.7,2.34 22.52,2.34
S$4184
  Bottom 0: 22.52,2.34 22.59,2.35
S$4185
  Bottom 0: 22.59,2.35 22.65,2.37
S$4186
  Bottom 0: 22.65,2.37 22.71,2.39
S$4187
  Bottom 0: 22.71,2.39 22.78,2.43
S$4188
  Bottom 0: 22.78,2.43 22.83,2.47
S$4189
  Bottom 0: 22.83,2.47 29.97,9.61
S$4190
  Bottom 0: 29.97,9.61 32.76,9.61
S$4191
  Bottom 0: 32.76,9.61 32.48,9.46
S$4192
  Bottom 0: 32.48,9.46 32.13,9.17
S$4193
  Bottom 0: 32.13,9.17 31.85,8.83
S$4194
  Bottom 0: 31.85,8.83 31.64,8.43
S$4195
  Bottom 0: 31.64,8.43 31.51,8
S$4196
  Bottom 0: 31.51,8 31.46,7.56
S$4197
  Bottom 0: 31.46,7.56 31.51,7.11
S$4198
  Bottom 0: 31.51,7.11 31.64,6.68
S$4199
  Bottom 0: 31.64,6.68 31.85,6.29
S$4200
  Bottom 0: 31.85,6.29 32.13,5.94
S$4201
  Bottom 0: 32.13,5.94 32.48,5.66
S$4202
  Bottom 0: 32.48,5.66 32.84,5.46
S$4203
  Bottom 0: 32.84,5.46 26.05,5.46
S$4204
  Bottom 0: 26.05,5.46 25.97,5.45
S$4205
  Bottom 0: 25.97,5.45 25.91,5.44
S$4206
  Bottom 0: 25.91,5.44 25.85,5.41
S$4207
  Bottom 0: 25.85,5.41 25.79,5.37
S$4208
  Bottom 0: 25.79,5.37 25.73,5.33
S$4209
  Bottom 0: 25.73,5.33 22.39,1.99
S$4210
  Bottom 0: 22.39,1.99 18.42,1.99
S$4211
  Bottom 0: 18.7,3.23 18.64,3.36
S$4212
  Bottom 0: 18.64,3.36 18.43,3.58
S$4213
  Bottom 0: 18.43,3.58 18.17,3.73
S$4214
  Bottom 0: 18.17,3.73 17.87,3.8
S$4215
  Bottom 0: 17.87,3.8 17.57,3.78
S$4216
  Bottom 0: 17.57,3.78 17.29,3.67
S$4217
  Bottom 0: 17.29,3.67 17.05,3.48
S$4218
  Bottom 0: 17.05,3.48 16.92,3.29
S$4219
  Bottom 0: 16.92,3.29 16.92,4.43
S$4220
  Bottom 0: 16.92,4.43 16.92,4.5
S$4221
  Bottom 0: 16.92,4.5 16.9,4.56
S$4222
  Bottom 0: 16.9,4.56 16.88,4.62
S$4223
  Bottom 0: 16.88,4.62 16.84,4.69
S$4224
  Bottom 0: 16.84,4.69 16.8,4.74
S$4225
  Bottom 0: 16.8,4.74 10.37,11.17
S$4226
  Bottom 0: 10.37,11.17 10.37,11.88
S$4227
  Bottom 0: 10.37,11.88 10.46,11.77
S$4228
  Bottom 0: 10.46,11.77 10.73,11.6
S$4229
  Bottom 0: 10.73,11.6 11.05,11.5
S$4230
  Bottom 0: 11.05,11.5 11.37,11.5
S$4231
  Bottom 0: 11.37,11.5 11.68,11.6
S$4232
  Bottom 0: 11.68,11.6 11.95,11.77
S$4233
  Bottom 0: 11.95,11.77 12.17,12.02
S$4234
  Bottom 0: 12.17,12.02 12.19,12.07
S$4235
  Bottom 0: 12.19,12.07 14.19,12.07
S$4236
  Bottom 0: 14.19,12.07 14.28,12.07
S$4237
  Bottom 0: 14.28,12.07 14.36,12.09
S$4238
  Bottom 0: 14.36,12.09 14.45,12.13
S$4239
  Bottom 0: 14.45,12.13 14.52,12.17
S$4240
  Bottom 0: 14.52,12.17 14.59,12.23
S$4241
  Bottom 0: 14.59,12.23 26.98,24.64
S$4242
  Bottom 0: 26.98,24.64 34.45,17.17
S$4243
  Bottom 0: 34.45,17.17 34.45,13.62
S$4244
  Bottom 0: 34.45,13.62 34.27,13.5
S$4245
  Bottom 0: 34.27,13.5 34.06,13.26
S$4246
  Bottom 0: 34.06,13.26 33.92,12.96
S$4247
  Bottom 0: 33.92,12.96 33.88,12.64
S$4248
  Bottom 0: 33.88,12.64 33.92,12.32
S$4249
  Bottom 0: 33.92,12.32 34.06,12.02
S$4250
  Bottom 0: 34.06,12.02 34.27,11.77
S$4251
  Bottom 0: 34.27,11.77 34.55,11.6
S$4252
  Bottom 0: 34.55,11.6 34.86,11.5
S$4253
  Bottom 0: 34.86,11.5 35.18,11.5
S$4254
  Bottom 0: 35.18,11.5 35.23,11.52
S$4255
  Bottom 0: 35.23,11.52 34.21,10.49
S$4256
  Bottom 0: 34.21,10.49 29.78,10.49
S$4257
  Bottom 0: 29.78,10.49 29.71,10.49
S$4258
  Bottom 0: 29.71,10.49 29.64,10.47
S$4259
